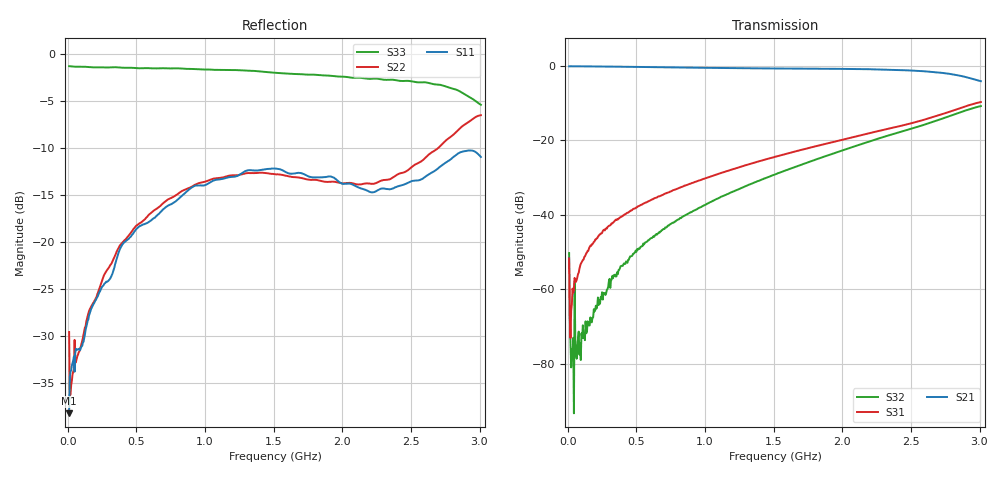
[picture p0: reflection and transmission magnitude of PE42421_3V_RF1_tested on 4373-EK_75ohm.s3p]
!Agilent Technologies,N5242A,MY49470268,A.09.90.13
!Agilent N5242A: A.09.90.13
!Date: Tuesday, October 06, 2015 13:31:27
!Correction: S11(Full 3 Port(1,2,3))
!S12(Full 3 Port(1,2,3))
!S13(Full 3 Port(1,2,3))
!S21(Full 3 Port(1,2,3))
!S22(Full 3 Port(1,2,3))
!S23(Full 3 Port(1,2,3))
!S31(Full 3 Port(1,2,3))
!S32(Full 3 Port(1,2,3))
!S33(Full 3 Port(1,2,3))
!S3P File: Measurements: <S11,S12,S13>,
!<S21,S22,S23>,
!<S31,S32,S33>:
# Hz S  dB  R 75
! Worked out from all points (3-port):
!   601 points, 10 MHz to 3.01 GHz, reference 75 ohm
!   strongest paths, dB at 10 MHz, 760 MHz, 1.51 GHz, 2.26 GHz, 3.01 GHz:
!     S21: -0.2, -0.5, -0.8, -1.0, -4.2
!     S31: -51.7, -33.6, -24.5, -17.6, -9.8
!     S32: -50.3, -42.2, -29.2, -19.6, -10.9
!   lowest |S11| = -38.2 dB at 10 MHz (marker M1), VSWR 1.02, Z = 76.8 - j0.509 ohm
!   |S11| at or under -10 dB: start of sweep to end of sweep
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1e7  -38.18 -15.6  -0.24 -1.9  -48.03 36.9
     -0.22 -1.7  -29.54 4.9  -49.00 -152.8
     -51.68 62.2  -50.25 -179.7  -1.30 178.7
3e7  -33.11 -28.6  -0.21 -4.5  -68.19 121.9
     -0.20 -4.4  -34.71 -32.3  -75.45 56.4
     -64.06 99.6  -76.00 17.6  -1.33 175.9
1.05e8  -31.03 -63.7  -0.23 -15.3  -53.05 81.5
        -0.22 -15.2  -30.54 -70.9  -72.41 114.8
        -52.45 81.7  -72.99 113.3  -1.35 165.6
3.3e8  -23.13 -130.9  -0.30 -47.6  -42.14 57.8
       -0.29 -47.5  -21.93 -124.8  -56.32 118.3
       -42.13 57.7  -57.02 117.8  -1.41 135.5
6.85e8  -16.67 172.4  -0.47 -98.0  -34.77 19.2
        -0.46 -97.8  -15.99 179.4  -44.04 80.9
        -34.78 19.3  -44.12 81.0  -1.51 88.6
1.12e9  -13.29 109.8  -0.66 -159.1  -28.77 -32.6
        -0.65 -159.0  -13.15 118.0  -35.17 23.8
        -28.74 -32.7  -35.11 23.7  -1.70 30.2
1.51e9  -12.17 54.6  -0.79 146.2  -24.48 -83.3
        -0.78 146.3  -12.78 67.2  -29.17 -29.6
        -24.47 -83.4  -29.21 -29.7  -2.00 -24.7
1.945e9  -13.21 -11.0  -0.88 84.0  -20.37 -144.1
         -0.88 84.1  -13.58 11.8  -23.44 -93.0
         -20.36 -144.1  -23.46 -93.0  -2.37 -91.1
2.385e9  -14.17 -93.7  -1.17 19.0  -16.52 149.6
         -1.16 19.2  -12.97 -48.9  -18.19 -164.0
         -16.52 149.8  -18.21 -163.9  -2.77 -159.4
3.01e9  -10.94 132.8  -4.20 -71.1  -9.79 24.0
        -4.20 -71.0  -6.51 -168.1  -10.86 65.0
        -9.79 24.2  -10.87 65.1  -5.40 120.1
